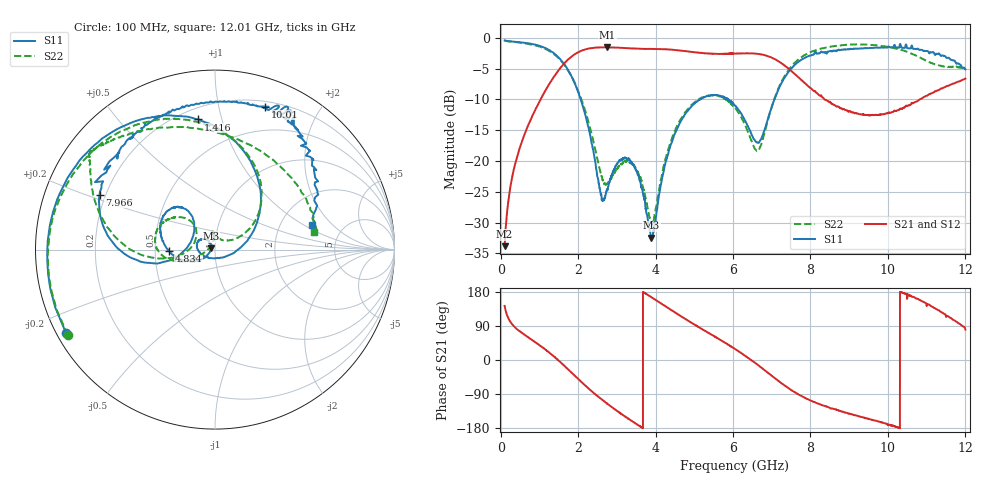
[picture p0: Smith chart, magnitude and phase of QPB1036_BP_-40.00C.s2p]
! TDS: K:\Engsetup\Winsaw\QPB1036_ALL
! Channel 1
! Ports=1 2
! seg 1=100.000000 1100.000000 101
! seg 2=1101.000000 1501.000000 401
! seg 3=1502.000000 2502.000000 101
! seg 4=2503.000000 3803.000000 1301
! seg 5=3804.000000 5004.000000 121
! seg 6=5005.000000 6005.000000 1001
! seg 7=6006.000000 8406.000000 241
! seg 8=8407.000000 10607.000000 2201
! seg 9=10608.000000 12008.000000 141
! Points=5609
! FailCode=0
! Topology=ALL_SE(12)
!VNA Cal loaded =QPB1036_ALL_-40C
!PS1(V)= 5.000
!PS(mA)= 0.800
!PS2(V)= 1.170
!PS(mA)= -0.100
!PS3(V)= 1.170
!PS(mA)= 0.100
!PS4(V)= 1.170
!PS(mA)= -0.100
!Temp (C)= -40.00
# MHz S DB R 50
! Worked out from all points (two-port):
!   5609 points, 100 MHz to 12.01 GHz, reference 50 ohm
!   highest |S21| = -1.53 dB at 2.75 GHz (marker M1); lowest = -33.8 dB at 100 MHz (marker M2)
!   |S21| within 3 dB of the highest: 1.588 GHz to 7.344 GHz (5.756 GHz wide, 129 % of centre)
!   lowest |S11| = -32.5 dB at 3.894 GHz (marker M3), VSWR 1.05, Z = 47.8 + j0.715 ohm
!   |S11| at or under -10 dB: 2.067 GHz to 5.145 GHz (3.077 GHz wide, 85.3 % of centre); 5.145488 GHz to 5.152685 GHz (7.197 MHz wide, 0.14 % of centre); 5.877 GHz to 7.07 GHz (1.194 GHz wide, 18.4 % of centre)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
!   |S22| runs from -30.4 to -0.5 dB; largest |S21 - S12| = 0.12
!   S11 on the Smith chart (normalised r, x): 100 MHz: 0.03, -0.26; 1.416 GHz: 0.27, +0.84; 4.834 GHz: 0.59, -0.01; 7.966 GHz: 0.18, +0.22; 10.01 GHz: 0.25, +1.38; 12.01 GHz: 2.96, +1.18
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100  -0.43 -150.8  -33.83 142.8  -33.78 143.2  -0.46 -149.9
730  -0.91 144.8  -13.90 58.3  -13.91 58.2  -1.04 148.5
1416  -2.72 97.5  -5.97 5.8  -5.95 5.6  -2.86 98.2
2092  -10.48 36.3  -2.08 -58.8  -2.11 -58.6  -10.10 39.4
2605  -25.80 -67.8  -1.54 -103.7  -1.56 -104.0  -22.43 43.8
2750  -24.54 -130.1  -1.53 -115.2  -1.56 -115.5  -23.56 71.2
3310  -19.87 149.9  -1.69 -155.8  -1.72 -155.8  -20.15 96.2
3894  -32.46 161.7  -1.82 165.7  -1.81 165.6  -30.11 136.9
4074  -26.15 -145.0  -1.83 153.7  -1.82 153.7  -25.37 -169.0
4834  -11.86 -178.0  -2.22 104.3  -2.21 104.1  -11.57 -168.3
5472  -9.29 147.2  -2.59 65.6  -2.58 65.0  -9.34 165.5
6056  -11.02 126.4  -2.57 28.9  -2.55 28.7  -11.39 137.8
6626  -16.96 154.3  -2.60 -11.7  -2.61 -11.9  -18.34 156.6
7116  -9.28 -167.0  -3.58 -50.6  -3.60 -50.6  -9.18 -172.3
7966  -2.94 154.6  -7.95 -105.2  -7.98 -105.2  -2.44 154.5
8046  -2.76 150.6  -8.38 -108.6  -8.38 -108.9  -2.21 152.6
8985  -1.84 108.6  -11.99 -141.1  -11.90 -141.0  -1.12 142.9
10012  -1.47 70.6  -12.16 -171.8  -12.29 -168.2  -1.52 133.6
10024  -1.41 69.6  -12.15 -171.7  -12.22 -168.9  -1.53 133.4
10978  -2.16 49.7  -9.46 150.6  -9.49 149.4  -3.68 90.2
11518  -3.26 35.7  -7.86 116.3  -7.90 118.3  -4.71 41.1
12008  -5.13 14.5  -6.63 80.1  -6.70 88.9  -4.96 8.8
